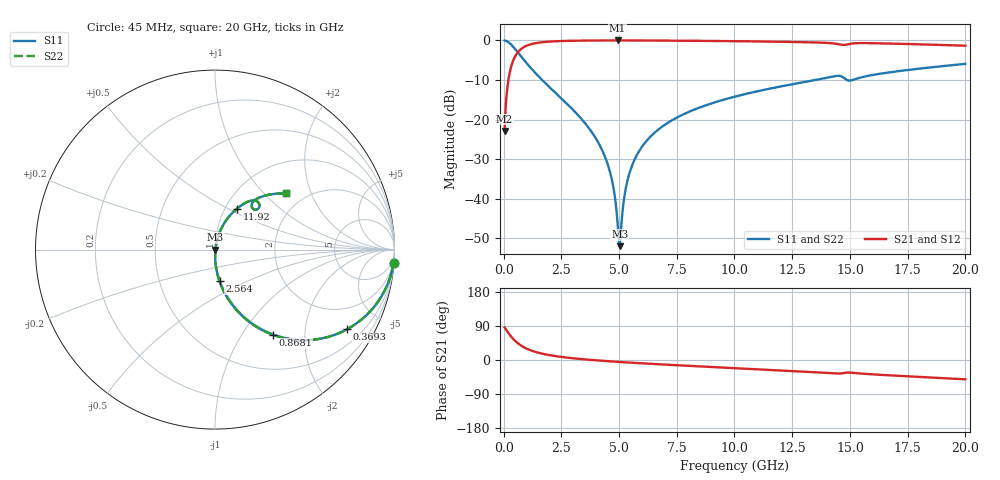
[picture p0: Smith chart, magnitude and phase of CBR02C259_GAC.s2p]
! S-parameter model data by Modelithics Inc.  support@modelithics.com 813-866-6335  Tampa FL USA
! S-Parameter data specifications:
! Substrate: 20-mil Rogers 4350B, substrate thickness, H=0.508mm, Dielectric constant, Er=3.75
! PCB Mounting Pad Footprint: Pad width, PadW=0.32mm , Pad length, PadL=0.37mm , Pad gap, PadG (edge-to-edge)=0.19mm , Reference planes=0.93mm apart
#  GHz  S  MA  R 50
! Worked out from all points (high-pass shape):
!   801 points, 45 MHz to 20 GHz, reference 50 ohm
!   highest |S21| = -0.02 dB at 4.934 GHz (marker M1); lowest = -22.9 dB at 45 MHz (marker M2)
!   |S21| within 3 dB of the highest: 615.7 MHz to end of sweep
!   lowest |S11| = -52.0 dB at 5.034 GHz (marker M3), VSWR 1.01, Z = 50.2 + j0.0383 ohm
!   |S11| at or under -10 dB: 1.67 GHz to 13.51 GHz (11.84 GHz wide, 156 % of centre); 14.87 GHz to 15.12 GHz (246.8 MHz wide, 1.65 % of centre)
!   |S22| runs from -52.0 to 0.0 dB; largest |S21 - S12| = 0
!   S11 on the Smith chart (normalised r, x): 45 MHz: 1, -28; 369.3 MHz: 0.98, -3.33; 868.1 MHz: 0.98, -1.38; 2.564 GHz: 0.99, -0.36; 11.92 GHz: 1.13, +0.56; 20 GHz: 1.61, +1.36
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0.045  0.9974 -4.2  0.07173 85.8  0.07173 85.8  0.9974 -4.2
0.219606  0.9433 -19.6  0.3316 70.4  0.3316 70.4  0.9433 -19.6
0.369269  0.8598 -31.0  0.5101 58.9  0.5101 58.9  0.8598 -31.0
0.868144  0.5728 -55.8  0.8186 34.0  0.8186 34.0  0.5728 -55.8
1.491737  0.3573 -70.4  0.9326 19.4  0.9326 19.4  0.3573 -70.4
2.564319  0.178 -81.8  0.9822 7.6  0.9822 7.6  0.178 -81.8
3.387462  0.1008 -86.5  0.9928 2.3  0.9928 2.3  0.1008 -86.5
4.036  0.05534 -88.7  0.9962 -1.0  0.9962 -1.0  0.05534 -88.7
4.484987  0.02863 -88.3  0.9972 -3.0  0.9972 -3.0  0.02863 -88.3
4.759369  0.01376 -84.1  0.9974 -4.1  0.9974 -4.1  0.01376 -84.1
4.933975  0.005071 -66.3  0.9975 -4.8  0.9975 -4.8  0.005071 -66.3
5.03375  0.00252 8.7  0.9975 -5.2  0.9975 -5.2  0.00252 8.7
5.283188  0.0131 72.8  0.9973 -6.2  0.9973 -6.2  0.0131 72.8
5.557569  0.0259 77.1  0.997 -7.2  0.997 -7.2  0.0259 77.1
6.0315  0.04695 77.8  0.9961 -8.9  0.9961 -8.9  0.04695 77.8
6.704981  0.07491 76.7  0.9943 -11.2  0.9943 -11.2  0.07491 76.7
8.051944  0.1261 73.1  0.9888 -15.5  0.9888 -15.5  0.1261 73.1
10.0225  0.1949 67.4  0.9771 -21.6  0.9771 -21.6  0.1949 67.4
11.91822  0.259 61.8  0.9614 -27.3  0.9614 -27.3  0.259 61.8
13.36496  0.3106 57.0  0.9439 -31.8  0.9439 -31.8  0.3106 57.0
16.68248  0.3934 48.6  0.9118 -40.4  0.9118 -40.4  0.3934 48.6
20  0.5053 38.2  0.8559 -51.0  0.8559 -51.0  0.5053 38.2
